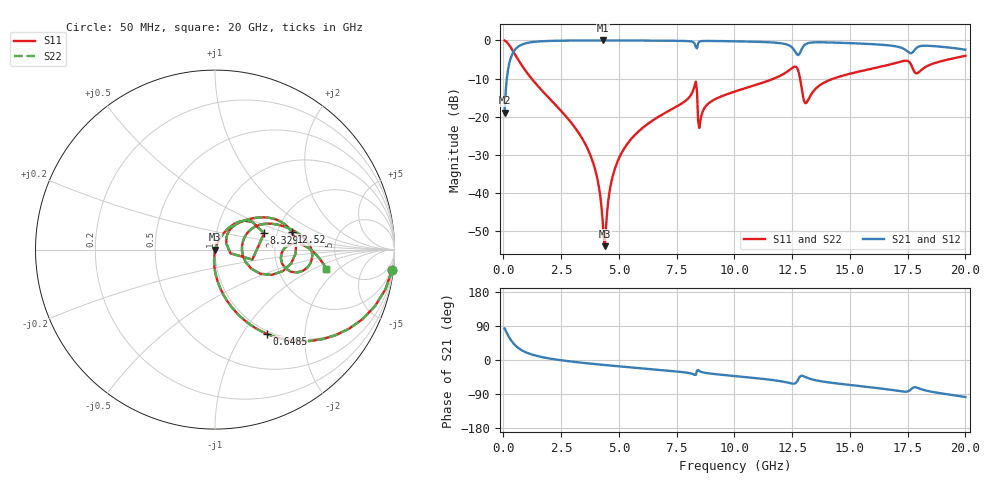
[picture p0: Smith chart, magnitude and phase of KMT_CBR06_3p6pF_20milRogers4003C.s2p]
! Data measured by Modelithics Inc. support@modelithics.com 813-866-6335
! KEMET CBR0603 3.6pF, Pad Width= 0.851mm, Pad Length= 0.64mm, Pad Gap= 0.62mm, 20mil Rogers 4003C substrate Data, January 2022
# hz S ma R 50
! 2 Port Network Data from SP1.SP block
! freq  magS11  angS11  magS21  angS21  magS12  angS12  magS22  angS22
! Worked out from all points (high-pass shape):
!   401 points, 50 MHz to 20 GHz, reference 50 ohm
!   highest |S21| = -0.02 dB at 4.289 GHz (marker M1); lowest = -18.9 dB at 50 MHz (marker M2)
!   |S21| within 3 dB of the highest: 435.4 MHz to 12.64 GHz (12.2 GHz wide, 187 % of centre); 12.85 GHz to 17.52 GHz (4.669 GHz wide, 30.7 % of centre)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
!   lowest |S11| = -53.9 dB at 4.389 GHz (marker M3), VSWR 1.00, Z = 50.2 + j0.0189 ohm
!   |S11| at or under -10 dB: 1.217 GHz to 11.71 GHz (10.49 GHz wide, 162 % of centre); 12.84 GHz to 14.29 GHz (1.448 GHz wide, 10.7 % of centre)
!   |S22| runs from -53.9 to -0.1 dB; largest |S21 - S12| = 0
!   S11 on the Smith chart (normalised r, x): 50 MHz: 1, -17; 648.5 MHz: 0.96, -1.29; 8.329 GHz: 1.71, +0.34; 12.52 GHz: 2.39, +0.58; 20 GHz: 3.88, -1.35
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5e7  0.9935 -6.7  0.1133 83.3  0.1133 83.3  0.9935 -6.7
2.99375e8  0.8244 -35.3  0.5653 54.6  0.5653 54.6  0.8244 -35.3
6.485e8  0.5517 -58.4  0.8332 31.5  0.8332 31.5  0.5517 -58.4
1.4465e9  0.2617 -78.9  0.9639 10.8  0.9639 10.8  0.2617 -78.9
3.391625e9  0.05295 -95.4  0.9968 -7.2  0.9968 -7.2  0.05295 -95.4
3.990125e9  0.0193 -95.5  0.9978 -10.9  0.9978 -10.9  0.0193 -95.5
4.289375e9  0.00458 -78.3  0.9979 -12.7  0.9979 -12.7  0.00458 -78.3
4.389125e9  0.002021 5.3  0.9979 -13.3  0.9979 -13.3  0.002021 5.3
4.688375e9  0.01474 67.3  0.9977 -15.0  0.9977 -15.0  0.01474 67.3
5.0375e9  0.03021 69.2  0.9973 -16.9  0.9973 -16.9  0.03021 69.2
6.73325e9  0.1008 62.5  0.9921 -26.0  0.9921 -26.0  0.1008 62.5
8.32925e9  0.2892 18.5  0.8143 -39.1  0.8143 -39.1  0.2892 18.5
8.52875e9  0.08957 45.1  0.9737 -30.5  0.9737 -30.5  0.08957 45.1
1.0025e10  0.2144 46.6  0.9723 -42.3  0.9723 -42.3  0.2144 46.6
1.251875e10  0.4389 13.0  0.7937 -62.4  0.7937 -62.4  0.4389 13.0
1.2818e10  0.3458 -24.1  0.6693 -45.3  0.6693 -45.3  0.3458 -24.1
1.306738e10  0.1504 -1.6  0.8845 -44.7  0.8845 -44.7  0.1504 -1.6
1.336662e10  0.2055 27.5  0.9393 -51.3  0.9393 -51.3  0.2055 27.5
1.670825e10  0.4814 9.9  0.8589 -78.1  0.8589 -78.1  0.4814 9.9
1.745638e10  0.5422 -5.6  0.7334 -83.5  0.7334 -83.5  0.5422 -5.6
1.790525e10  0.3706 -3.8  0.806 -73.0  0.806 -73.0  0.3706 -3.8
2e10  0.6283 -9.7  0.7549 -97.6  0.7549 -97.6  0.6283 -9.7
